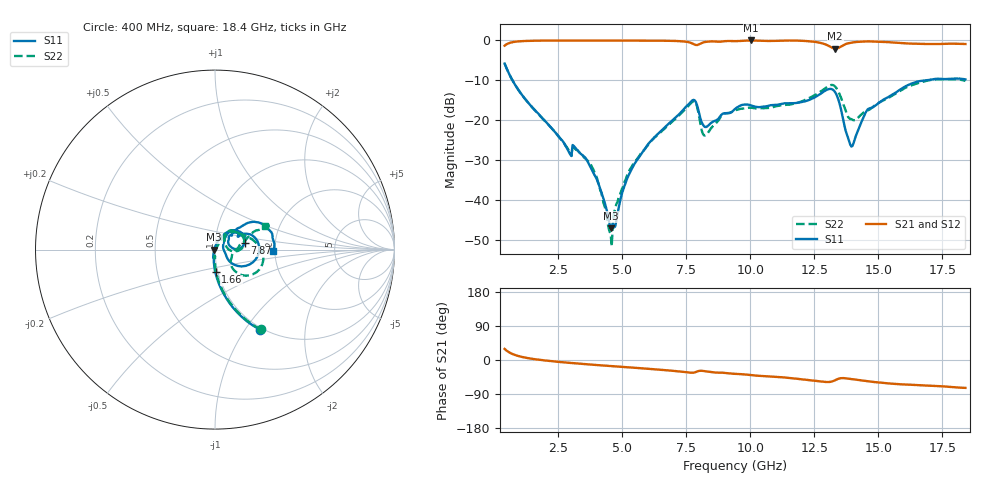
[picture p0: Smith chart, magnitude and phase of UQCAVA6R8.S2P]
!  Part Number  UQCAVA6R8	Mounting Orientation: Horizontal
!  Description: RF capacitors
!  Application: Coupling, Bypass, Tuning, DC Block
!  Filters, Matching
# GHZ S DB R 50
! Freq  |S11|  S11 Ph  |S21|  S21 Ph  |S12|  S12 Ph  |S22|  S22 Ph
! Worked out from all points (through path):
!   401 points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, 400 MHz to 18.4 GHz, reference 50 ohm
!   highest |S21| = -0.03 dB at 10.03 GHz (marker M1); lowest = -2.1 dB at 13.31 GHz (marker M2)
!   group delay of S21, straight-line fit = 12.5 ps
!   lowest |S11| = -47.1 dB at 4.54 GHz (marker M3), VSWR 1.01, Z = 49.6 - j0.112 ohm
!   |S11| at or under -10 dB: 705.5 MHz to 16.91 GHz (16.2 GHz wide, 184 % of centre)
!   |S22| runs from -51.6 to -5.8 dB; largest |S21 - S12| = 0.0021
!   S11 on the Smith chart (normalised r, x): 400 MHz: 0.97, -1.17; 1.66 GHz: 0.97, -0.25; 7.87 GHz: 1.39, +0.10; 18.4 GHz: 1.96, -0.04
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0.4  -5.82 -60.7  -1.33 29.3  -1.33 29.3  -5.81 -60.3
0.85  -11.56 -78.0  -0.32 12.3  -0.33 12.3  -11.57 -77.2
1.66  -18.03 -88.6  -0.09 1.4  -0.09 1.4  -18.04 -87.6
2.92  -28.06 -99.7  -0.05 -7.4  -0.05 -7.4  -27.64 -89.8
3.145  -26.77 -99.4  -0.06 -8.8  -0.06 -8.8  -27.12 -91.8
3.415  -28.64 -101.1  -0.05 -10.3  -0.06 -10.3  -28.78 -92.4
3.955  -34.25 -112.0  -0.06 -13.0  -0.06 -13.0  -33.59 -99.5
4.54  -47.07 -165.3  -0.05 -16.0  -0.05 -15.9  -48.42 -30.5
4.72  -46.64 105.2  -0.05 -16.9  -0.05 -16.9  -42.26 27.6
5.26  -33.59 80.5  -0.05 -19.5  -0.05 -19.5  -32.85 54.2
6.43  -23.20 65.3  -0.09 -25.4  -0.09 -25.4  -23.41 56.1
7.87  -15.45 12.2  -1.16 -31.8  -1.16 -31.8  -15.76 8.8
8.23  -21.72 19.9  -0.41 -29.7  -0.40 -29.6  -23.85 24.9
9.4  -17.19 42.6  -0.20 -36.5  -0.19 -36.5  -17.55 52.6
10.03  -16.32 29.2  -0.03 -39.8  -0.02 -39.8  -16.89 47.3
12.415  -14.61 28.5  -0.31 -54.0  -0.30 -54.0  -14.07 20.8
13.315  -13.02 -18.2  -2.09 -53.3  -2.09 -53.4  -11.59 -28.7
13.945  -26.61 7.2  -0.60 -50.3  -0.60 -50.3  -19.74 -25.7
14.575  -17.36 47.5  -0.26 -55.9  -0.25 -55.9  -17.59 5.9
15.43  -14.03 41.1  -0.48 -62.0  -0.47 -62.0  -14.29 20.2
16.555  -10.29 26.9  -0.86 -66.4  -0.85 -66.4  -10.69 24.2
18.4  -9.78 -1.4  -0.92 -73.6  -0.91 -73.7  -10.16 25.5
